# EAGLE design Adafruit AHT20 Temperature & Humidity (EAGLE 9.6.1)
COMPANY: ADAFRUIT INDUSTRIES; DRAWN: KTOWN; REV: A
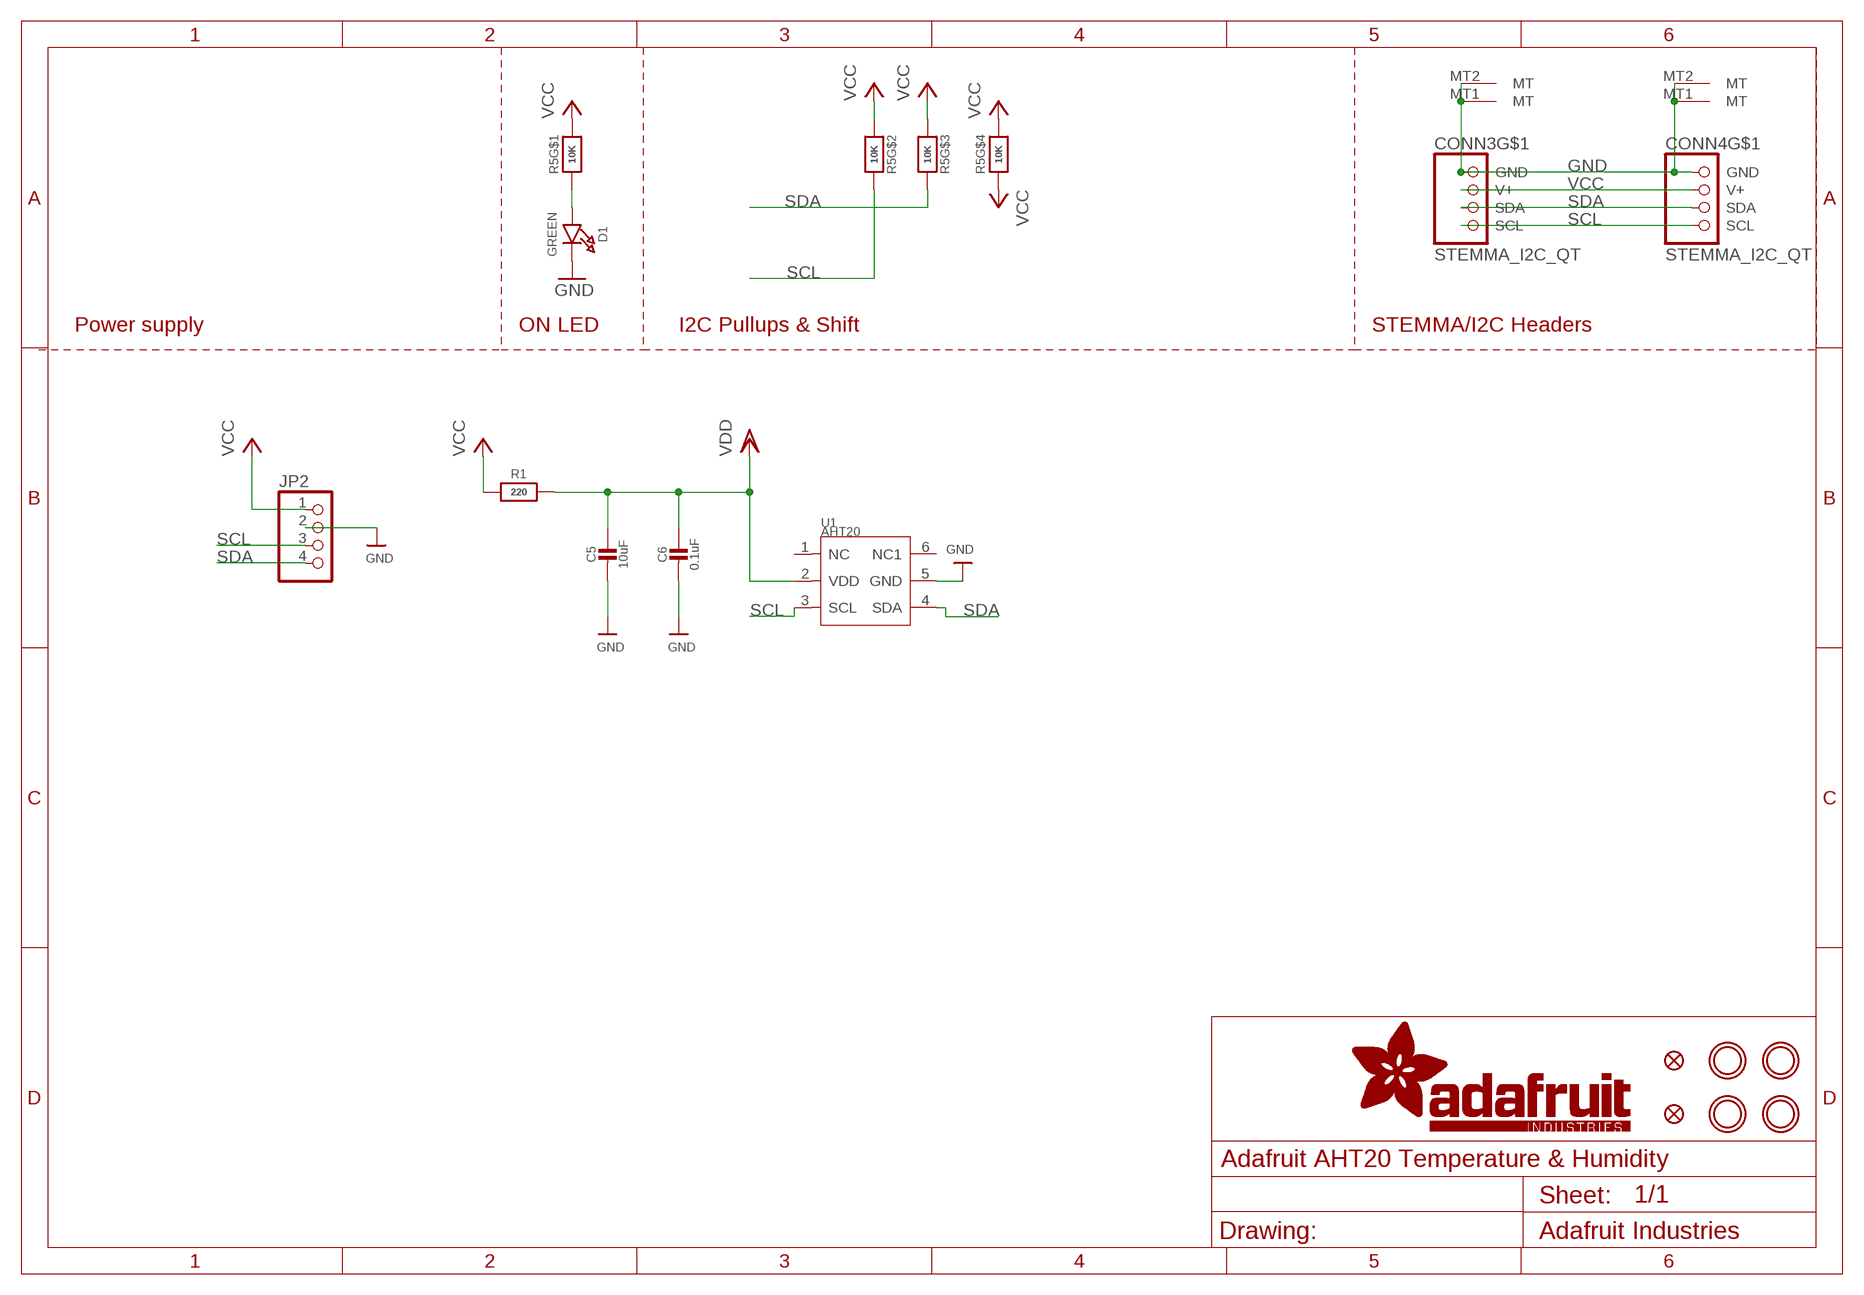
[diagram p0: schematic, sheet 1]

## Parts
C5  10uF  CAP_CERAMIC0805-NOOUTLINE  [0805-NO]
C6  0.1uF  CAP_CERAMIC0603_NO  [0603-NO]
CONN3  STEMMA_I2C_QT  [JST_SH4]
CONN4  STEMMA_I2C_QT  [JST_SH4]
D1  GREEN  LED0603_NOOUTLINE  [CHIPLED_0603_NOOUTLINE]
FID3  FIDUCIAL_1MM  [FIDUCIAL_1MM]
FID4  FIDUCIAL_1MM  [FIDUCIAL_1MM]
JP2  HEADER-1X476MIL  [1X04_ROUND_76]
R1  220  RESISTOR_0603_NOOUT  [0603-NO]
R5  10K  RESISTOR_4PACK  [RESPACK_4X0603]
U1  AHT20  SENSOR-AHT20  [SNR6-1.0-3X3X1MM]
U$19  MOUNTINGHOLE2.5  [MOUNTINGHOLE_2.5_PLATED]
U$20  MOUNTINGHOLE2.5  [MOUNTINGHOLE_2.5_PLATED]
U$22  MOUNTINGHOLE2.5  [MOUNTINGHOLE_2.5_PLATED]
U$25  MOUNTINGHOLE2.5  [MOUNTINGHOLE_2.5_PLATED]

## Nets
GND: C5.2 C6.2 CONN3.1(GND) CONN3.MT1(MT) CONN3.MT2(MT) CONN4.1(GND) CONN4.MT1(MT) CONN4.MT2(MT) D1.C JP2.2 U1.5(GND)
N$1: D1.A R5.1
SCL: CONN3.4(SCL) CONN4.4(SCL) JP2.3 R5.7 U1.3(SCL)
SDA: CONN3.3(SDA) CONN4.3(SDA) JP2.4 R5.6 U1.4(SDA)
VCC [highpower]: CONN3.2(V+) CONN4.2(V+) JP2.1 R1.1 R5.2 R5.3 R5.4 R5.5 R5.8
VDD: C5.1 C6.1 R1.2 U1.2(VDD)
Unconnected: U1.1(NC) U1.6(NC1)

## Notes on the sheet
- Power supply | ON LED | I2C Pullups & Shift | STEMMA/I2C Headers

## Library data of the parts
C5 C6 = microbuilder:CAP_CERAMIC: Ceramic Capacitors
CONN3 CONN4 = microbuilder:STEMMA_I2C
D1 = microbuilder:LED: LED
FID3 FID4 = microbuilder:FIDUCIAL: Fiducial Alignment Points; BOM: EXCLUDE
JP2 = microbuilder:HEADER-1X4: PIN HEADER
R1 = microbuilder:RESISTOR: Resistors
R5 = microbuilder:RESISTOR_4PACK: Resistor Packs (4 resistors) 4 x 0603 10K 1/16W - Digikey: YC164J-10KCT-ND
U1 = Longan-IC:SENSOR-AHT20
U$19 U$20 U$22 U$25 = microbuilder:MOUNTINGHOLE: Mounting Hole; BOM: EXCLUDE

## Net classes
1 highpower: width 0.305 mm, drill 0.483 mm
2 lowpower: width 0.254 mm, drill 0.483 mm

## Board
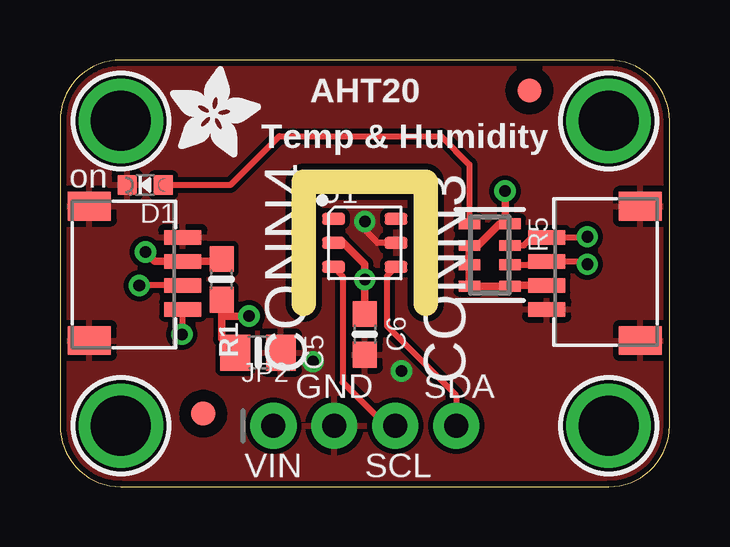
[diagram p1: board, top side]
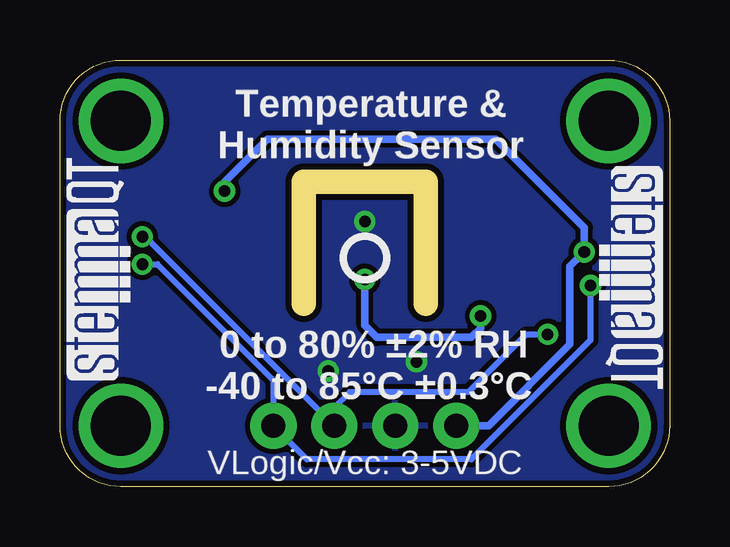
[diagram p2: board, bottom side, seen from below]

Size 25.4 x 17.78 mm. Coordinates in mm from the lower left corner, seen from the top.
Outline: 10.16,7.62 10.16,12.7 15.24,12.7 15.24,7.62
Outline: 0,15.24 0,2.54 arc90 2.54,0 22.86,0 arc90 25.4,2.54 25.4,15.24 arc90 22.86,17.78 2.54,17.78 arc90 0,15.24
Copper layers (1*16): Top 0.035mm / dielectric 1.5mm / Bottom 0.035mm
Design rules "adafruit": minimum track width 8mil, minimum drill 15.5mil, track to track 8mil, track to pad 8mil, pad to pad 8mil, via to via 8mil, smd to smd 8mil, copper to edge 10mil, drill to drill 8mil, minimum pad ring 10mil, minimum via ring 8mil, stop-mask expansion 2mil, vias tented up to drill 20mil, thermal gap 10mil

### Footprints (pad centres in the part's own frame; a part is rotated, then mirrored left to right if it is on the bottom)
0805-NO = smd 1.24 x 1.5: 1 -0.95,0; 2 0.95,0
0603-NO = smd 1.075 x 1: 1 -0.85,0; 2 0.85,0
JST_SH4 = smd 0.6 x 1.55: 1 -1.5,2.514; 2 -0.5,2.514; 3 0.5,2.514; 4 1.5,2.514 | smd 1.2 x 1.8: MT1 -2.8,-1.386; MT2 2.8,-1.386
CHIPLED_0603_NOOUTLINE = smd 0.8 x 0.8: A 0,-0.75; C 0,0.75
FIDUCIAL_1MM = smd 1 x 1: 1 0,0
1X04_ROUND_76 = drill 1 pad 1.93: 1 -3.81,0; 2 -1.27,0; 3 1.27,0; 4 3.81,0
RESPACK_4X0603 = smd 0.45 x 0.9: 1 -1.3,-0.85; 2 -0.4,-0.85; 3 0.4,-0.85; 4 1.3,-0.85; 5 1.3,0.85; 6 0.4,0.85; 7 -0.4,0.85; 8 -1.3,0.85
SNR6-1.0-3X3X1MM = smd 0.95 x 0.5: 1 -1.3,1; 2 -1.3,0; 3 -1.3,-1; 4 1.3,-1; 5 1.3,0; 6 1.3,1
MOUNTINGHOLE_2.5_PLATED = drill 2.5 pad 3.2: P$1 0,0

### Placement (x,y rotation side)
C5  8.26,5.59 0 top
C6  12.7,6.35 270 top
CONN3  22.8,8.89 90 top
CONN4  2.6,8.89 270 top
D1  3.56,12.57 90 top
FID3  5.97,3.05 0 top
FID4  19.56,16.51 0 top
JP2  12.7,2.54 0 top
R1  6.73,8.64 270 top
R5  17.91,9.65 270 top
U1  12.7,10.16 0 top
U$19  2.54,15.24 0 top
U$20  22.86,15.24 0 top
U$22  2.54,2.54 0 top
U$25  22.86,2.54 0 top
U$28  [ADAFRUIT_3.5MM]  4.57,13.72 0 top
U$29  [PCBFEAT-REV-040]  12.7,9.53 0 bottom
U$30  [STEMMAQT]  22.48,4.45 90 bottom
U$31  [STEMMAQT]  2.92,13.34 270 bottom

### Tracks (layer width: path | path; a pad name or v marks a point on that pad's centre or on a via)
GND  (via drill 0.48)
  Top 0.254: U1.5 13.24,10.16 12.7,10.7 v12.7,11.05
  other vias: 14.22,4.83 10.54,5.21
  pour Top: 0,17.78 25.4,17.78 25.4,0 0,0
  pour Bottom: 0,17.78 25.4,17.78 25.4,0 0,0
N$1
  Top 0.254: D1.A 7.11,12.57 9.14,14.61 15.88,14.61 17.06,13.42 R5.1
SCL  (via drill 0.48)
  Top 0.254: JP2.3 13.59,2.54 11.78,4.35 11.78,8.78 U1.3 | R5.7 19.32,10.05 19.66,10.39 CONN3.4 21.95,10.39 v21.97,10.41 | CONN4.4 5.1,7.38 5.1,6.37 v5.08,6.35
  Bottom 0.254: v21.97,10.41 21.84,10.41 JP2.3 13.97,3.3 13.34,3.94 8.38,3.94 5.97,6.35 v5.08,6.35
SDA  (via drill 0.48)
  Top 0.254: U1.4 13.62,8.78 13.62,6.7 16.51,3.81 JP2.4 | R5.6 19.54,9.25 19.68,9.4 CONN3.3 21.85,9.39 v21.97,9.27 | CONN4.3 v3.31,8.39 v3.3,8.38
  Bottom 0.254: v21.97,9.27 21.35,9.27 16.51,4.43 JP2.4 15.11,1.14 8.26,1.14 3.3,6.1 v3.3,8.38
VCC  (via drill 0.48)
  Top 0.305: CONN3.2 18.8,8.39 R5.5 R5.4 R5.3 R5.2 17.42,10.05 18.32,10.95 18.54,10.95 | R5.8 18.54,10.95 | R1.1 6.63,9.39 CONN4.2 3.94,9.39 v3.56,9.78 | v18.54,12.32 18.54,10.95
  Bottom 0.305: JP2.1 7.54,2.54 4.15,5.93 4.15,9.18 v3.56,9.78 3.56,10.79 7.24,14.48 16.76,14.48 18.54,12.7 v18.54,12.32
VDD  (via drill 0.48)
  Top 0.305: C5.1 6.73,6.16 R1.2 6.73,7.11 v7.87,7.11 | C6.1 v12.7,8.64 12.7,9.27 11.81,10.16 U1.2
  Bottom 0.305: v7.87,7.11 7.87,6.6 8.26,6.22 12.19,6.22 12.7,6.73 v12.7,8.64

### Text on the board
tPlace: AHT20 | Temp & Humidity | on | GND | SDA | VIN | SCL
bPlace: Temperature & / Humidity Sensor | 0 to 80% ±2% RH / -40 to 85°C ±0.3°C | VLogic/Vcc: 3-5VDC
